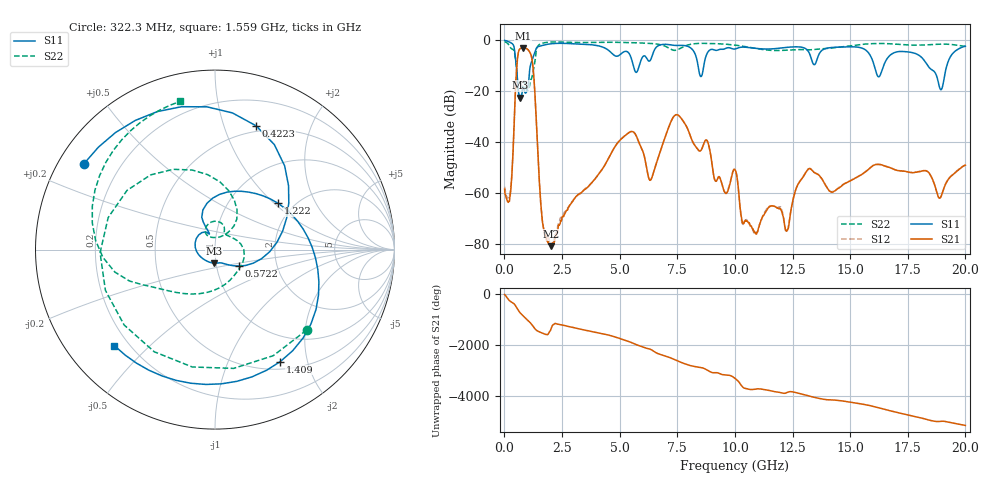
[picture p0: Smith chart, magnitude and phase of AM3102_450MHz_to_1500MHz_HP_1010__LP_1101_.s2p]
!Agilent Technologies,E8364B,MY43040894,A.07.50.67
!Agilent E8364B: A.07.50.67
!Date: Thursday, January 11, 2018 06:20:58
!Correction: S11(Full 2 Port(1,2))
!S21(Full 2 Port(1,2))
!S12(Full 2 Port(1,2))
!S22(Full 2 Port(1,2))
!S2P File: Measurements: S11, S21, S12, S22:
# Hz S  dB  R 50
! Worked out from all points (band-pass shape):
!   1601 points, 10 MHz to 20 GHz, reference 50 ohm
!   highest |S21| = -2.97 dB at 809.6 MHz (marker M1); lowest = -80.7 dB at 2.021 GHz (marker M2)
!   |S21| within 3 dB of the highest: 584.3 MHz to 1.163 GHz (578.9 MHz wide, 66.3 % of centre)
!   lowest |S11| = -22.4 dB at 684.7 MHz (marker M3), VSWR 1.16, Z = 48.9 - j7.42 ohm
!   |S11| at or under -10 dB: 518.8 MHz to 1.127 GHz (608.1 MHz wide, 73.9 % of centre); 16.05 GHz to 16.45 GHz (401 MHz wide, 2.47 % of centre); 18.37 GHz to 19.19 GHz (820.4 MHz wide, 4.37 % of centre)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
!   |S22| runs from -23.4 to -0.5 dB; largest |S21 - S12| = 0.0018
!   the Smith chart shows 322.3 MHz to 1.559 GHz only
!   S11 on the Smith chart (normalised r, x): 322.3 MHz: 0.07, +0.29; 422.3 MHz: 0.44, +1.29; 572.2 MHz: 1.28, -0.24; 1.222 GHz: 1.66, +1.06; 1.409 GHz: 0.60, -1.57; 1.559 GHz: 0.15, -0.39
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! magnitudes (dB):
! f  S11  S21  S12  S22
! 10 MHz  -0.1  -58.3  -57.4  -0.5
! 322.3 MHz  -1.2  -53.3  -52.6  -3.4
! 422.3 MHz  -2.8  -32.9  -32.9  -4.1
! 572.2 MHz  -15.8  -6.9  -6.9  -17.1
! 684.7 MHz  -22.4  -3.3  -3.3  -23.4
! 809.6 MHz  -18.6  -3.0  -3.0  -17.0
! 1.222 GHz  -7.2  -8.9  -8.9  -13.4
! 1.409 GHz  -2.8  -36.2  -36.1  -3.1
! 1.559 GHz  -2.2  -61.5  -61.9  -1.4
! 2.021 GHz  -1.4  -80.7  -80.4  -0.7
! 3.346 GHz  -1.5  -59.7  -59.6  -0.9
! 5.432 GHz  -5.5  -36.0  -36.0  -0.9
! 6.682 GHz  -2.1  -45.8  -45.8  -1.6
! 7.494 GHz  -2.0  -29.2  -29.2  -3.8
! 9.58 GHz  -3.3  -59.9  -59.7  -1.5
! 10.01 GHz  -3.4  -50.7  -50.6  -1.9
! 10.89 GHz  -3.1  -75.5  -75.4  -3.2
! 12.27 GHz  -2.8  -74.6  -74.7  -3.9
! 13.34 GHz  -7.9  -50.9  -50.9  -3.7
! 16.68 GHz  -6.4  -49.8  -49.7  -1.3
! 18.94 GHz  -19.4  -61.4  -61.4  -1.5
! 20 GHz  -2.3  -49.0  -48.9  -2.3
